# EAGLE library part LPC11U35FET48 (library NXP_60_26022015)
32-bit ARM Cortex-M0 microcontroller; up to 128 kB flash; up to 12 kB SRAM and 4 kB EEPROM; USB device; USART The LPC11U3x are a ARM Cortex-M0 based, low-cost 32-bit MCU family, designed for 8/16-bit microcontroller applications, offering performance, low power, simple instruction set and memory addressing together with reduced code size compared to existing 8/16-bit architectures. The LPC11U3x operate at CPU frequencies of up to 50 MHz. Equipped with a highly flexible and configurable Full Speed USB 2.0 device controller, the LPC11U3x brings unparalleled design flexibility and seamless integration to today’s demanding connectivity solutions. The peripheral complement of the LPC11U3x includes up to 128 kB of flash memory, up to 12 kB of SRAM data memory and 4 kB EEPROM, one Fast-mode Plus I 2 C-bus interface, one RS-485/EIA-485 USART with support for synchronous mode and smart card interface, two SSP interfaces, four general purpose counter/timers, a 10-bit ADC, and up to 54 general purpose I/O pins. AAL Eindhoven MK
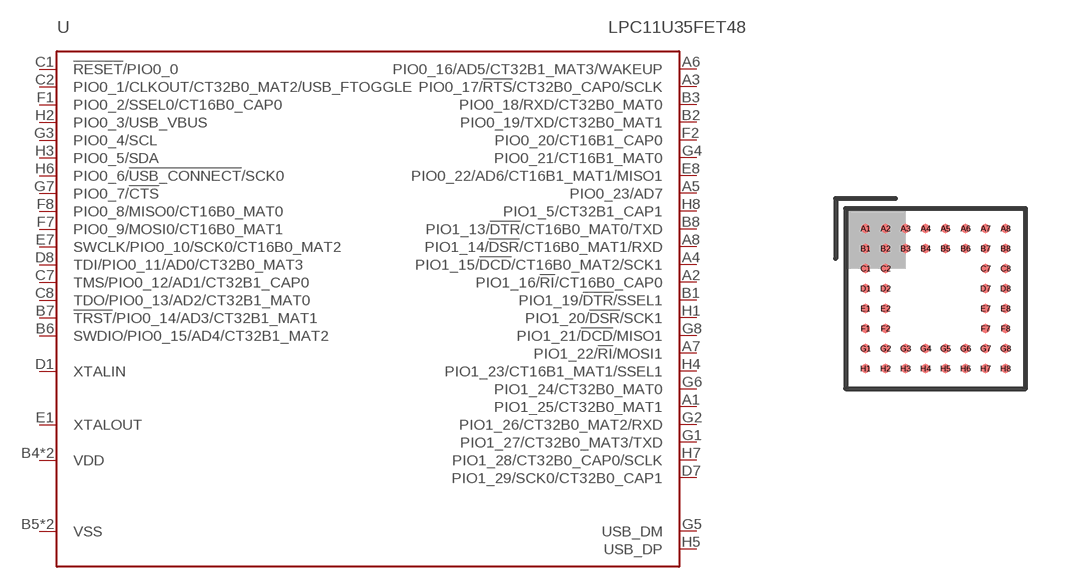
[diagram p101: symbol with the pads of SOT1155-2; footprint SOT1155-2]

Designator prefix U

## LPC11U35FET48/501 (FLASH: 64kB; GPIO: 40; SRAM: 12kB)  [SOT1155-2]
A1  PIO1_25/CT32B0_MAT1
A2  PIO1_16/!RI!/CT16B0_CAP0
A3  PIO0_17/!RTS!/CT32B0_CAP0/SCLK
A4  PIO1_15/!DCD!/CT16B0_MAT2/SCK1
A5  PIO0_23/AD7
A6  PIO0_16/AD5/CT32B1_MAT3/WAKEUP
A7  PIO1_22/!RI!/MOSI1
A8  PIO1_14/!DSR!/CT16B0_MAT1/RXD
B1  PIO1_19/!DTR!/SSEL1
B2  PIO0_19/TXD/CT32B0_MAT1
B3  PIO0_18/RXD/CT32B0_MAT0
B4  VDD  pwr
B5  VSS  pwr
B6  SWDIO/PIO0_15/AD4/CT32B1_MAT2
B7  !TRST!/PIO0_14/AD3/CT32B1_MAT1
B8  PIO1_13/!DTR!/CT16B0_MAT0/TXD
C1  !RESET!/PIO0_0
C2  PIO0_1/CLKOUT/CT32B0_MAT2/USB_FTOGGLE
C7  TMS/PIO0_12/AD1/CT32B1_CAP0
C8  TDO/PIO0_13/AD2/CT32B1_MAT0
D1  XTALIN  in
D2  VSS  pwr
D7  PIO1_29/SCK0/CT32B0_CAP1
D8  TDI/PIO0_11/AD0/CT32B0_MAT3
E1  XTALOUT  out
E2  VDD  pwr
E7  SWCLK/PIO0_10/SCK0/CT16B0_MAT2
E8  PIO0_22/AD6/CT16B1_MAT1/MISO1
F1  PIO0_2/SSEL0/CT16B0_CAP0
F2  PIO0_20/CT16B1_CAP0
F7  PIO0_9/MOSI0/CT16B0_MAT1
F8  PIO0_8/MISO0/CT16B0_MAT0
G1  PIO1_27/CT32B0_MAT3/TXD
G2  PIO1_26/CT32B0_MAT2/RXD
G3  PIO0_4/SCL
G4  PIO0_21/CT16B1_MAT0
G5  USB_DM
G6  PIO1_24/CT32B0_MAT0
G7  PIO0_7/!CTS!
G8  PIO1_21/!DCD!/MISO1
H1  PIO1_20/!DSR!/SCK1
H2  PIO0_3/USB_VBUS
H3  PIO0_5/SDA
H4  PIO1_23/CT16B1_MAT1/SSEL1
H5  USB_DP
H6  PIO0_6/!USB_CONNECT!/SCK0
H7  PIO1_28/CT32B0_CAP0/SCLK
H8  PIO1_5/CT32B1_CAP1

## Footprint SOT1155-2 (pad centres in mm)
SOT1155-2 TFBGA48: plastic thin fine-pitch ball grid array package; 48 balls; body 4.5 x 4.5 x 0.7 mm JEDEC: -- IEC: -- JEITA: --
smd 0.225 x 0.225: A1 -1.75,1.75; A2 -1.25,1.75; A3 -0.75,1.75; A4 -0.25,1.75; A5 0.25,1.75; A6 0.75,1.75; A7 1.25,1.75; A8 1.75,1.75; B1 -1.75,1.25; B2 -1.25,1.25; B3 -0.75,1.25; B4 -0.25,1.25; B5 0.25,1.25; B6 0.75,1.25; B7 1.25,1.25; B8 1.75,1.25; C1 -1.75,0.75; C2 -1.25,0.75; C7 1.25,0.75; C8 1.75,0.75; D1 -1.75,0.25; D2 -1.25,0.25; D7 1.25,0.25; D8 1.75,0.25; E1 -1.75,-0.25; E2 -1.25,-0.25; E7 1.25,-0.25; E8 1.75,-0.25; F1 -1.75,-0.75; F2 -1.25,-0.75; F7 1.25,-0.75; F8 1.75,-0.75; G1 -1.75,-1.25; G2 -1.25,-1.25; G3 -0.75,-1.25; G4 -0.25,-1.25; G5 0.25,-1.25; G6 0.75,-1.25; G7 1.25,-1.25; G8 1.75,-1.25; H1 -1.75,-1.75; H2 -1.25,-1.75; H3 -0.75,-1.75; H4 -0.25,-1.75; H5 0.25,-1.75; H6 0.75,-1.75; H7 1.25,-1.75; H8 1.75,-1.75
